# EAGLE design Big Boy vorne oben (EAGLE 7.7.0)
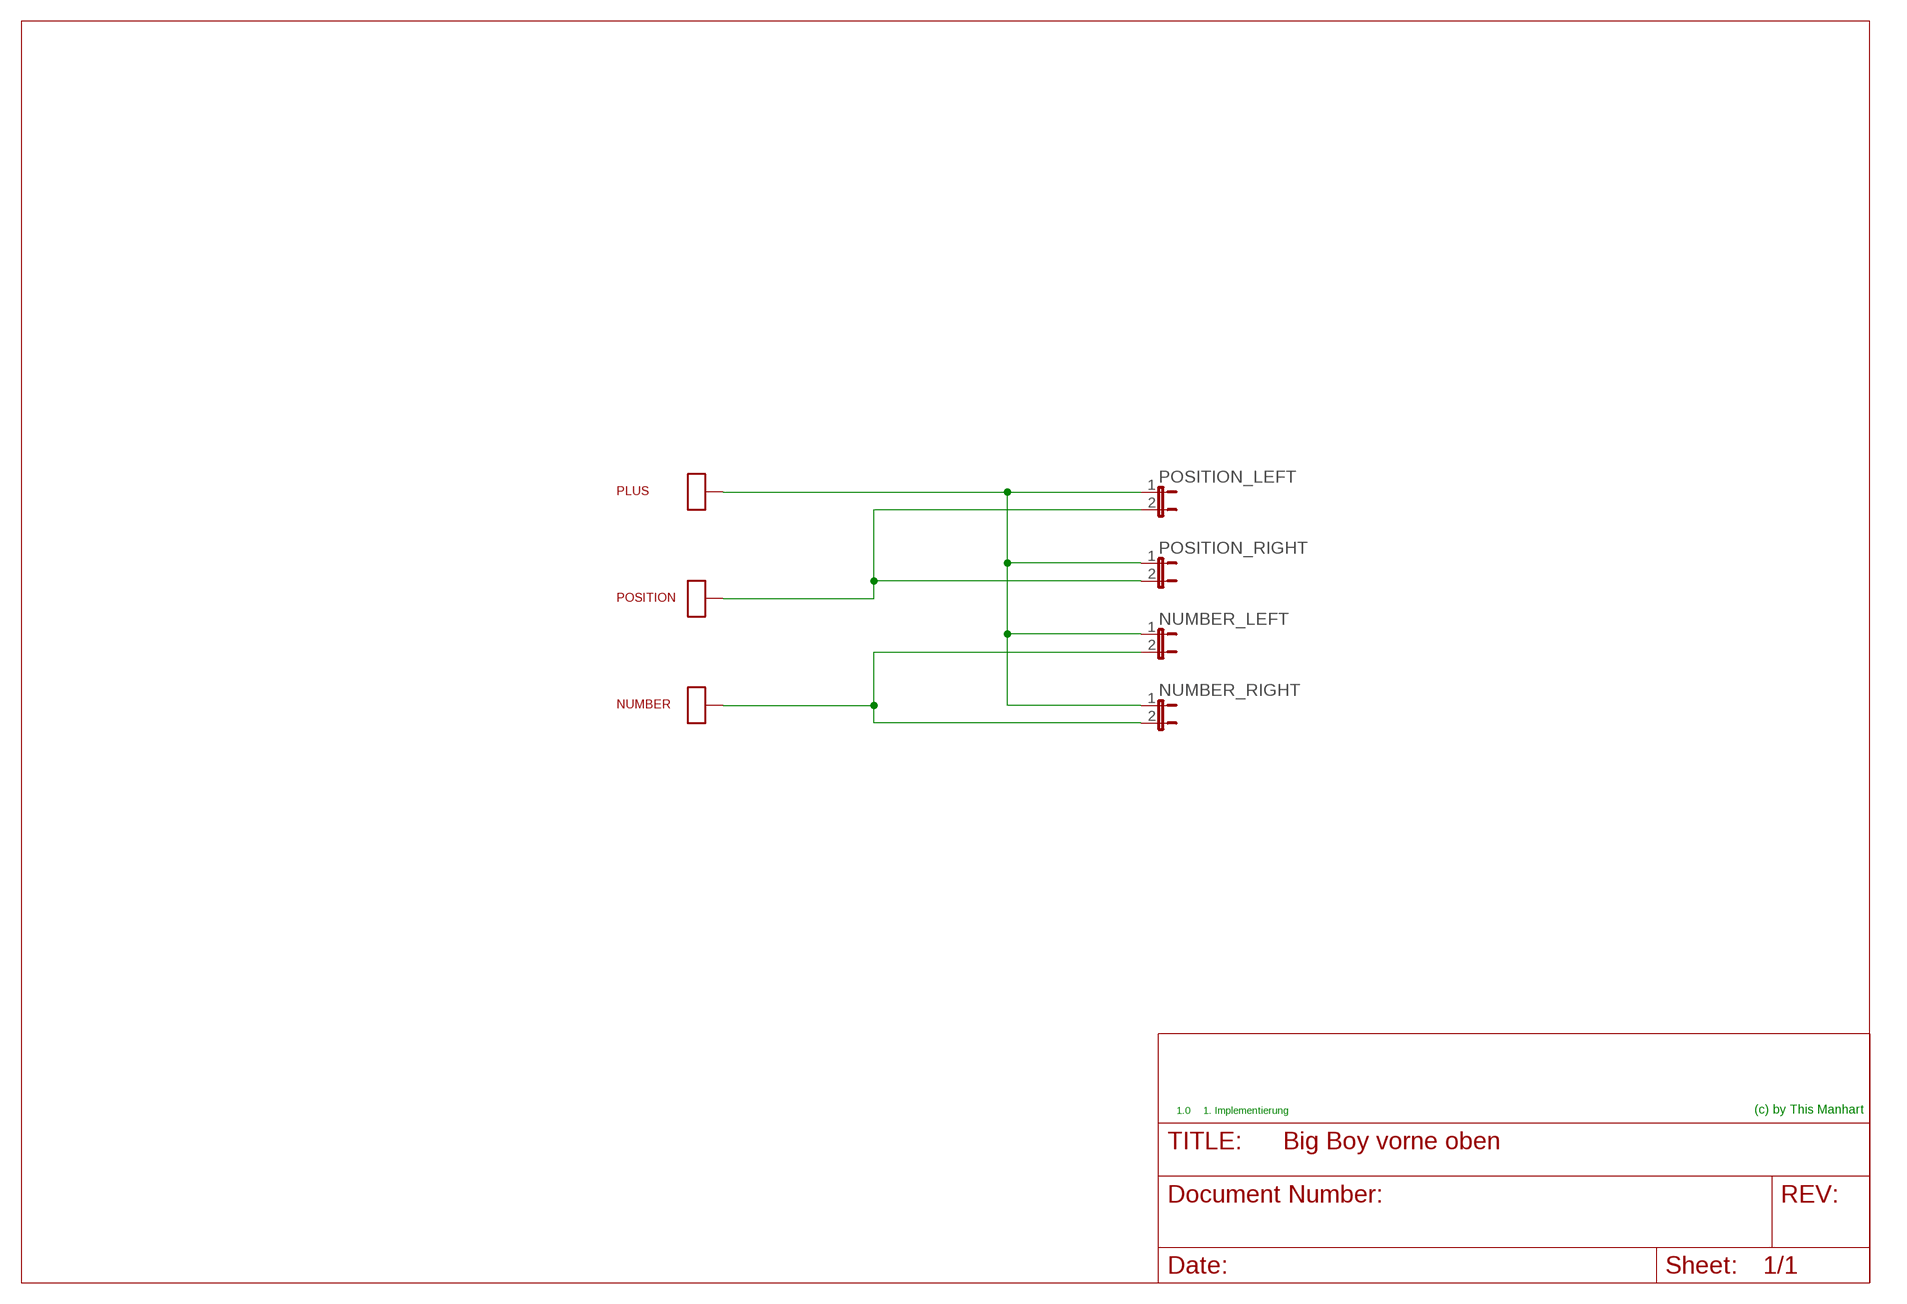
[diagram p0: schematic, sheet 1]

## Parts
NUMBER  SMD_LOETPAD  [SMD_LOETPAD_XL]
NUMBER_LEFT  JUMPER_2P  [JUMPER_2P_2.54_OHNE]
NUMBER_RIGHT  JUMPER_2P  [JUMPER_2P_2.54_OHNE]
PLUS  SMD_LOETPAD  [SMD_LOETPAD_XL]
POSITION  SMD_LOETPAD  [SMD_LOETPAD_XL]
POSITION_LEFT  JUMPER_2P  [JUMPER_2P_2.54_OHNE]
POSITION_RIGHT  JUMPER_2P  [JUMPER_2P_2.54_OHNE]

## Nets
N$1: NUMBER_LEFT.1 NUMBER_RIGHT.1 PLUS.P$1 POSITION_LEFT.1 POSITION_RIGHT.1
N$3: POSITION.P$1 POSITION_LEFT.2 POSITION_RIGHT.2
N$4: NUMBER.P$1 NUMBER_LEFT.2 NUMBER_RIGHT.2

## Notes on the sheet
- 1.0 | 1. Implementierung | (c) by This Manhart

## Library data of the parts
NUMBER PLUS POSITION = 0_mm:SMD_LOETPAD
NUMBER_LEFT NUMBER_RIGHT POSITION_LEFT POSITION_RIGHT = 0_mm:JUMPER_2P

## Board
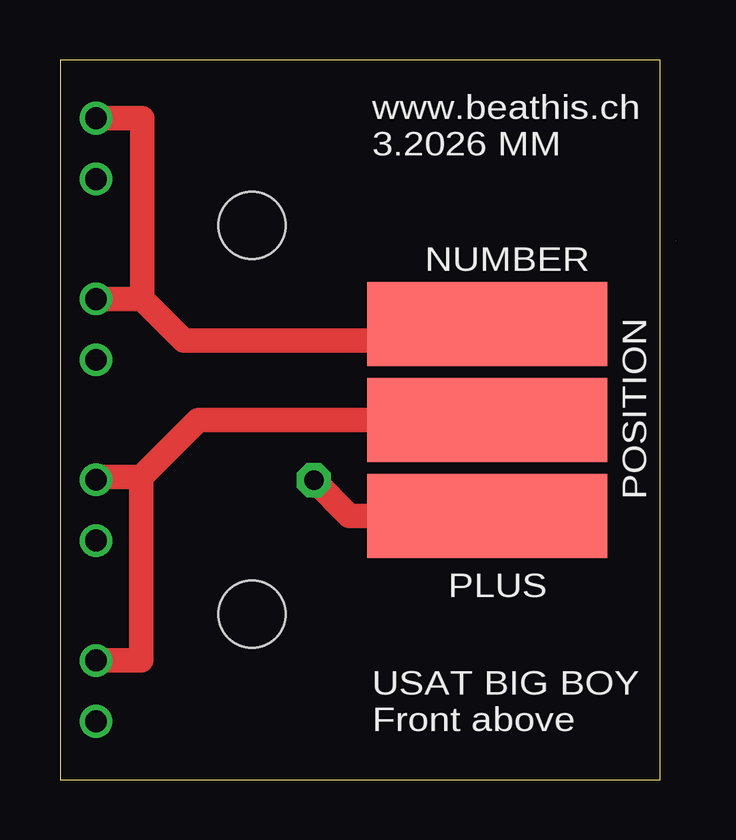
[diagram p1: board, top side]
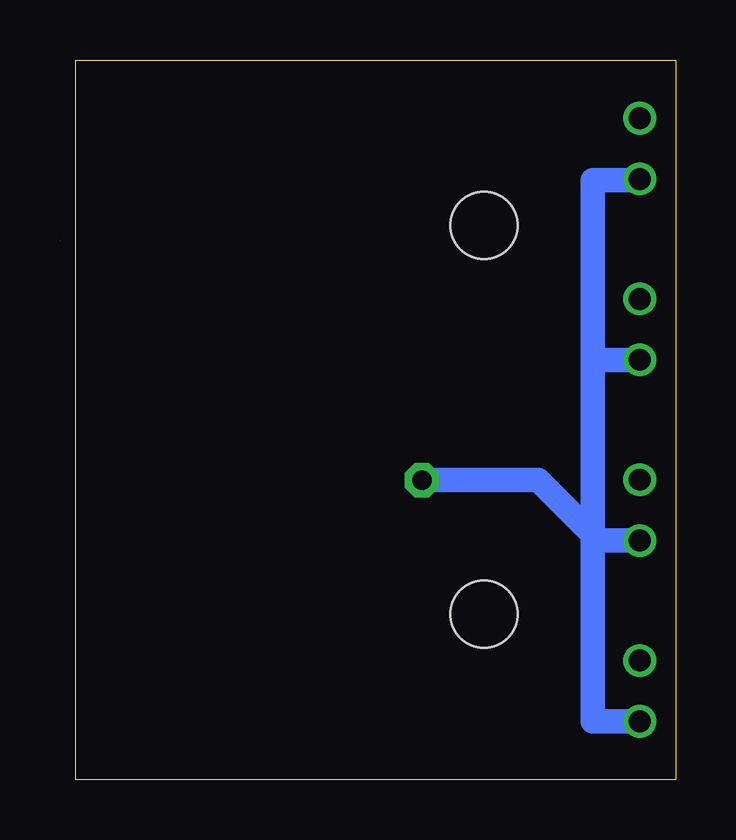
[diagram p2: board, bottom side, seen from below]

Size 25.66 x 30 mm. Coordinates in mm from the lower left corner, seen from the top.
Outline: 25.65,22.45 25.66,22.45
Outline: 25,0 25,30 0,30 0,0 25,0
Copper layers (1*16): Top 0.035mm / dielectric 1.5mm / Bottom 0.035mm
Design rules "pcb-pool": minimum track width 6mil, minimum drill 12mil, track to track 6mil, track to pad 6mil, pad to pad 6mil, via to via 6mil, smd to smd 8mil, copper to edge 40mil, drill to drill 20mil, minimum pad ring 8mil, minimum via ring 8mil, stop-mask expansion 6mil, vias tented up to drill 0mil, thermal gap 10mil
Holes 2.8 mm at 8,6.9 8,23.1

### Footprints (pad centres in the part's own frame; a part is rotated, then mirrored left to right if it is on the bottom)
SMD_LOETPAD_XL = smd 10 x 3.5: P$1 0,0
JUMPER_2P_2.54_OHNE = drill 0.914: 1 -2.54,0; 2 0,0

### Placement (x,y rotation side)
NUMBER  17.8,19 0 top
NUMBER_LEFT  1.5,27.58 90 top
NUMBER_RIGHT  1.5,20.04 90 top
PLUS  17.8,11 180 top
POSITION  17.8,15 0 top
POSITION_LEFT  1.5,12.5 90 top
POSITION_RIGHT  1.5,4.96 90 top

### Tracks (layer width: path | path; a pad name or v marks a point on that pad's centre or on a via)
N$1  (via drill 0.8 pad 1.42)
  Top 1.016: PLUS.P$1 12.06,11 v10.58,12.48
  Bottom 1.016: POSITION_RIGHT.1 3.47,2.42 3.47,10.01 | 3.47,10.01 3.47,10.22 | 3.47,10.22 3.47,17.44 | 3.47,17.44 3.47,25 1.5,25 NUMBER_LEFT.1 | v10.58,12.48 5.73,12.48 3.47,10.22 | POSITION_LEFT.1 3.42,9.96 3.47,10.01 | NUMBER_RIGHT.1 3.41,17.5 3.47,17.44
N$3
  Top 1.016: POSITION_RIGHT.2 3.38,4.96 3.38,12.61 | 3.38,12.61 1.5,12.61 POSITION_LEFT.2 | POSITION.P$1 5.77,15 3.38,12.61
N$4
  Top 1.016: NUMBER_LEFT.2 3.43,27.58 3.43,20.04 | NUMBER_RIGHT.2 3.43,20.04 | 3.43,20.04 3.43,20.03 | 3.43,20.04 5.16,18.31 17.31,18.31 17.8,18.8 NUMBER.P$1

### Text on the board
tNames: www.beathis.ch / 3.2026 MM | NUMBER | POSITION | PLUS | USAT BIG BOY / Front above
